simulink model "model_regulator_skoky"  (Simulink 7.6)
settings: Solver=ode45  StartTime=0.0  StopTime=150  RelTol=1e-3
undefined symbols (not defined in the file or in its folder): D, I

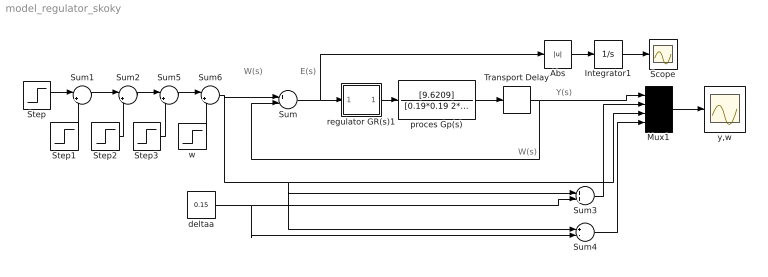
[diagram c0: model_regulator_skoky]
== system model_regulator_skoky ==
  note: W(s)
  note: Y(s)
  note: E(s)
  note: W(s)
  Abs : Abs
  Integrator1 : Integrator
  Mux1 : Mux
  Scope : Scope
  Step : Step  Time=0  After=11  SampleTime=0
  Step1 : Step  Time=30  After=30  SampleTime=0
  Step2 : Step  Time=60  After=-11  SampleTime=0
  Step3 : Step  Time=90  After=-25  SampleTime=0
  Sum : Sum  Inputs=+-
  Sum{1..2,5..6} (4 alike) : Sum  Inputs=|++
  Sum3 : Sum
  Sum4 : Sum  Inputs=+-
  Transport Delay : TransportDelay  DelayTime=0.4
  deltaa : Constant  Value=0.15
  proces Gp(s) : TransferFcn  Numerator=[9.6209]  Denominator=[0.19*0.19 2*0.19 1]
  regulator GR(s)1 : Subsystem  mask(PID Controller){P=0.11217,  I=0.11217/0.77427,  D=0.11217*0.14103}
      mask prompts: P "Proportional";  I "Integral";  D "Derivative"
      mask help: Enter expressions for proportional, integral, and derivative terms. P+I/s+Ds
  w : Step  Time=120  After=17  SampleTime=0
  y,w : Scope
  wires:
  Sum6/1 -> Sum/1, Sum3/1, Sum4/1, Mux1/3
  proces Gp(s)/1 -> Transport Delay/1
  Mux1/1 -> y,w/1
  deltaa/1 -> Sum3/2, Sum4/2
  Sum3/1 -> Mux1/2
  Sum4/1 -> Mux1/4
  Transport Delay/1 -> Sum/2, Mux1/1
  Step1/1 -> Sum1/2
  Step/1 -> Sum1/1
  Step2/1 -> Sum2/2
  Step3/1 -> Sum5/2
  Sum2/1 -> Sum5/1
  Sum1/1 -> Sum2/1
  Sum5/1 -> Sum6/1
  w/1 -> Sum6/2
  Integrator1/1 -> Scope/1
  Abs/1 -> Integrator1/1
  regulator GR(s)1/1(Out_1) -> proces Gp(s)/1
  Sum/1 -> regulator GR(s)1/1(In_1), Abs/1

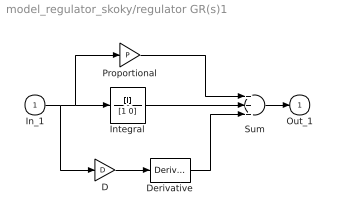
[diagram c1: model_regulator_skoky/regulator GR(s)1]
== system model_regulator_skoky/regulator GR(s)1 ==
  In_1 : Inport
  D : Gain  Gain=D
  Derivative : Derivative
  Integral : TransferFcn  Numerator=[I]  Denominator=[1 0]
  Proportional : Gain  Gain=P
  Sum : Sum  Inputs=+++
  Out_1 : Outport
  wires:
  D/1 -> Derivative/1
  Sum/1 -> Out_1/1
  In_1/1 -> D/1, Proportional/1, Integral/1
  Derivative/1 -> Sum/3
  Integral/1 -> Sum/2
  Proportional/1 -> Sum/1
